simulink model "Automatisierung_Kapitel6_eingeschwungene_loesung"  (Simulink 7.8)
settings: Solver=ode45  StartTime=0.0  StopTime=50  MaxStep=0.2  RelTol=1e-3
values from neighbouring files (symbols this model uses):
  A = A0*A1*A2    [Automatisierung_Kapitel6.m]
  A0 = 10    [Automatisierung_Kapitel6.m]
  p = (p1+p2)*180/pi    [Automatisierung_Kapitel6.m]
  TA4 = 0.6    [Automatisierung_Kapitel6.m]
  w0 = 1    [Automatisierung_Kapitel6.m]
libraries: cstblocks x1

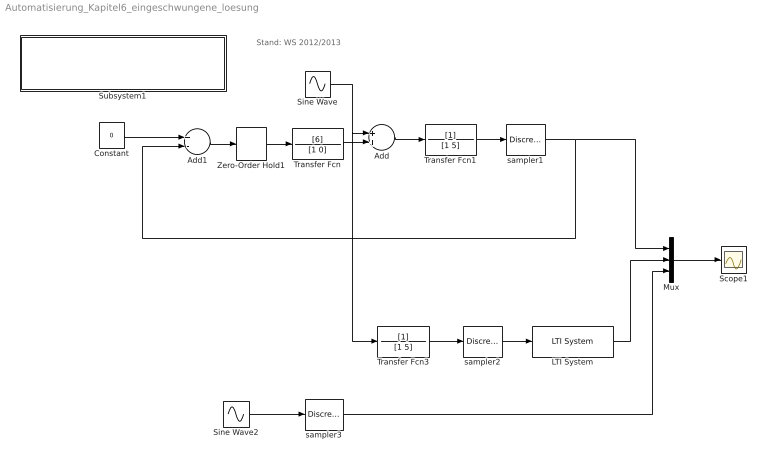
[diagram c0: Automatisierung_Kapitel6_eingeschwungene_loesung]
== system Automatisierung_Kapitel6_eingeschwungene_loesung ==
  note: Stand: WS 2012/2013
  Add : Sum
  Add1 : Sum  Inputs=+-
  Constant : Constant  Value=0
  LTI System : cstblocks/LTI System  sys=Tdyz  IC=[]
  Mux : Mux  Inputs=3
  Scope1 : Scope
  Sine Wave : Sin  Amplitude=A0  Frequency=w0  SampleTime=0
  Sine Wave2 : Sin  Amplitude=A  Frequency=2  Phase=p*pi/180  SampleTime=0
  Subsystem1 : Subsystem  Description=asas
  Transfer Fcn : TransferFcn  Numerator=[6]  Denominator=[1 0]
  Transfer Fcn1 : TransferFcn  Denominator=[1 5]
  Transfer Fcn3 : TransferFcn  Denominator=[1 5]
  Zero-Order Hold1 : ZeroOrderHold  SampleTime=TA4
  sampler1 : DiscreteTransferFcn  Denominator=[1]  SampleTime=TA4
  sampler2 : DiscreteTransferFcn  Denominator=[1]  SampleTime=TA4
  sampler3 : DiscreteTransferFcn  Denominator=[1]  SampleTime=TA4
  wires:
  Add/1 -> Transfer Fcn1/1
  Transfer Fcn1/1 -> sampler1/1
  Zero-Order Hold1/1 -> Transfer Fcn/1
  Transfer Fcn/1 -> Add/2
  Add1/1 -> Zero-Order Hold1/1
  sampler1/1 -> Add1/2, Mux/1
  Constant/1 -> Add1/1
  Transfer Fcn3/1 -> sampler2/1
  Mux/1 -> Scope1/1
  sampler2/1 -> LTI System/1
  Sine Wave2/1 -> sampler3/1
  sampler3/1 -> Mux/3
  LTI System/1 -> Mux/2
  Sine Wave/1 -> Transfer Fcn3/1, Add/1

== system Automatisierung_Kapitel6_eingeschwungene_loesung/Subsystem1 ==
